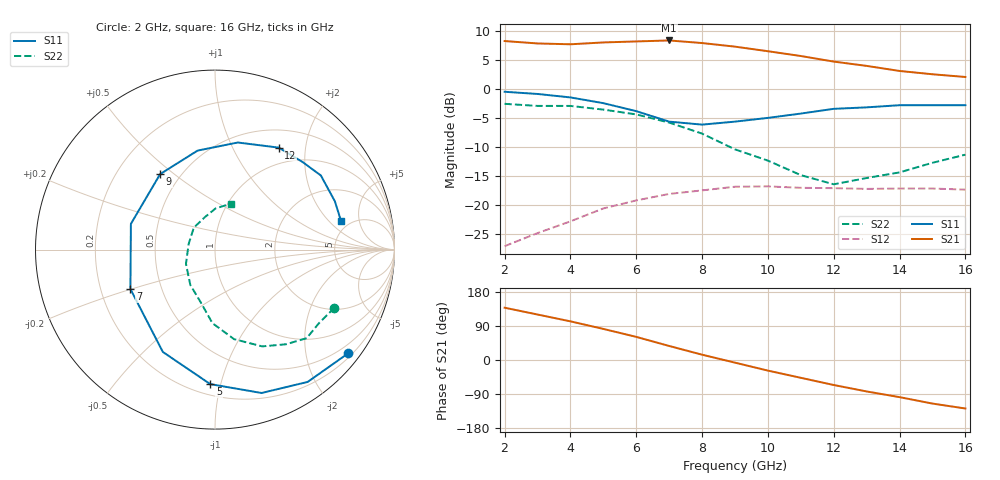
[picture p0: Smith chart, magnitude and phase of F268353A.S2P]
!ATF-26835
!S-PARAMETERS at Vds=3V  Id=10mA.  LAST UPDATED 07-22-92
# ghz s ma r 50
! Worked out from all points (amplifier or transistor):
!   15 points, 2 GHz to 16 GHz, reference 50 ohm
!   highest |S21| = 8.3 dB at 7 GHz (marker M1)
!   |S21| within 3 dB of that: start of sweep to 11.33 GHz
!   unconditionally stable (mu >= 1): 7.295 GHz to end of sweep
!   at 4 GHz: K = 0.59, MSG = 15.2 dB, |S12| = -22.9 dB
!   at 9 GHz: K = 1.07, MAG = 10.5 dB, |S12| = -16.9 dB
!   at 16 GHz: K = 1.31, MAG = 6.4 dB, |S12| = -17.4 dB
!   S11 on the Smith chart (normalised r, x): 2 GHz: 0.29, -2.88; 5 GHz: 0.27, -0.93; 7 GHz: 0.33, -0.20; 9 GHz: 0.39, +0.45; 12 GHz: 0.75, +1.54; 16 GHz: 4.18, +2.81
2  0.94 -38.0  2.57 138.0  0.044 60.0  0.74 -26.0
3  0.9 -55.0  2.45 120.0  0.057 51.0  0.71 -35.0
4  0.84 -72.0  2.41 102.0  0.072 44.0  0.71 -44.0
5  0.75 -92.0  2.5 82.0  0.093 30.0  0.66 -53.0
6  0.64 -117.0  2.55 61.0  0.109 15.0  0.6 -64.0
7  0.52 -155.0  2.6 37.0  0.124 5.0  0.51 -78.0
8  0.49 163.0  2.47 14.0  0.133 -12.0  0.41 -92.0
9  0.52 126.0  2.3 -7.0  0.143 -21.0  0.3 -106.0
10  0.56 100.0  2.1 -28.0  0.144 -32.0  0.24 -125.0
11  0.61 78.0  1.91 -47.0  0.14 -41.0  0.18 -154.0
12  0.67 58.0  1.71 -66.0  0.139 -49.0  0.15 168.0
13  0.69 45.0  1.57 -83.0  0.137 -61.0  0.17 134.0
14  0.72 35.0  1.42 -98.0  0.138 -66.0  0.19 107.0
15  0.72 22.0  1.33 -115.0  0.138 -77.0  0.23 89.0
16  0.72 13.0  1.26 -128.0  0.135 -85.0  0.27 71.0
